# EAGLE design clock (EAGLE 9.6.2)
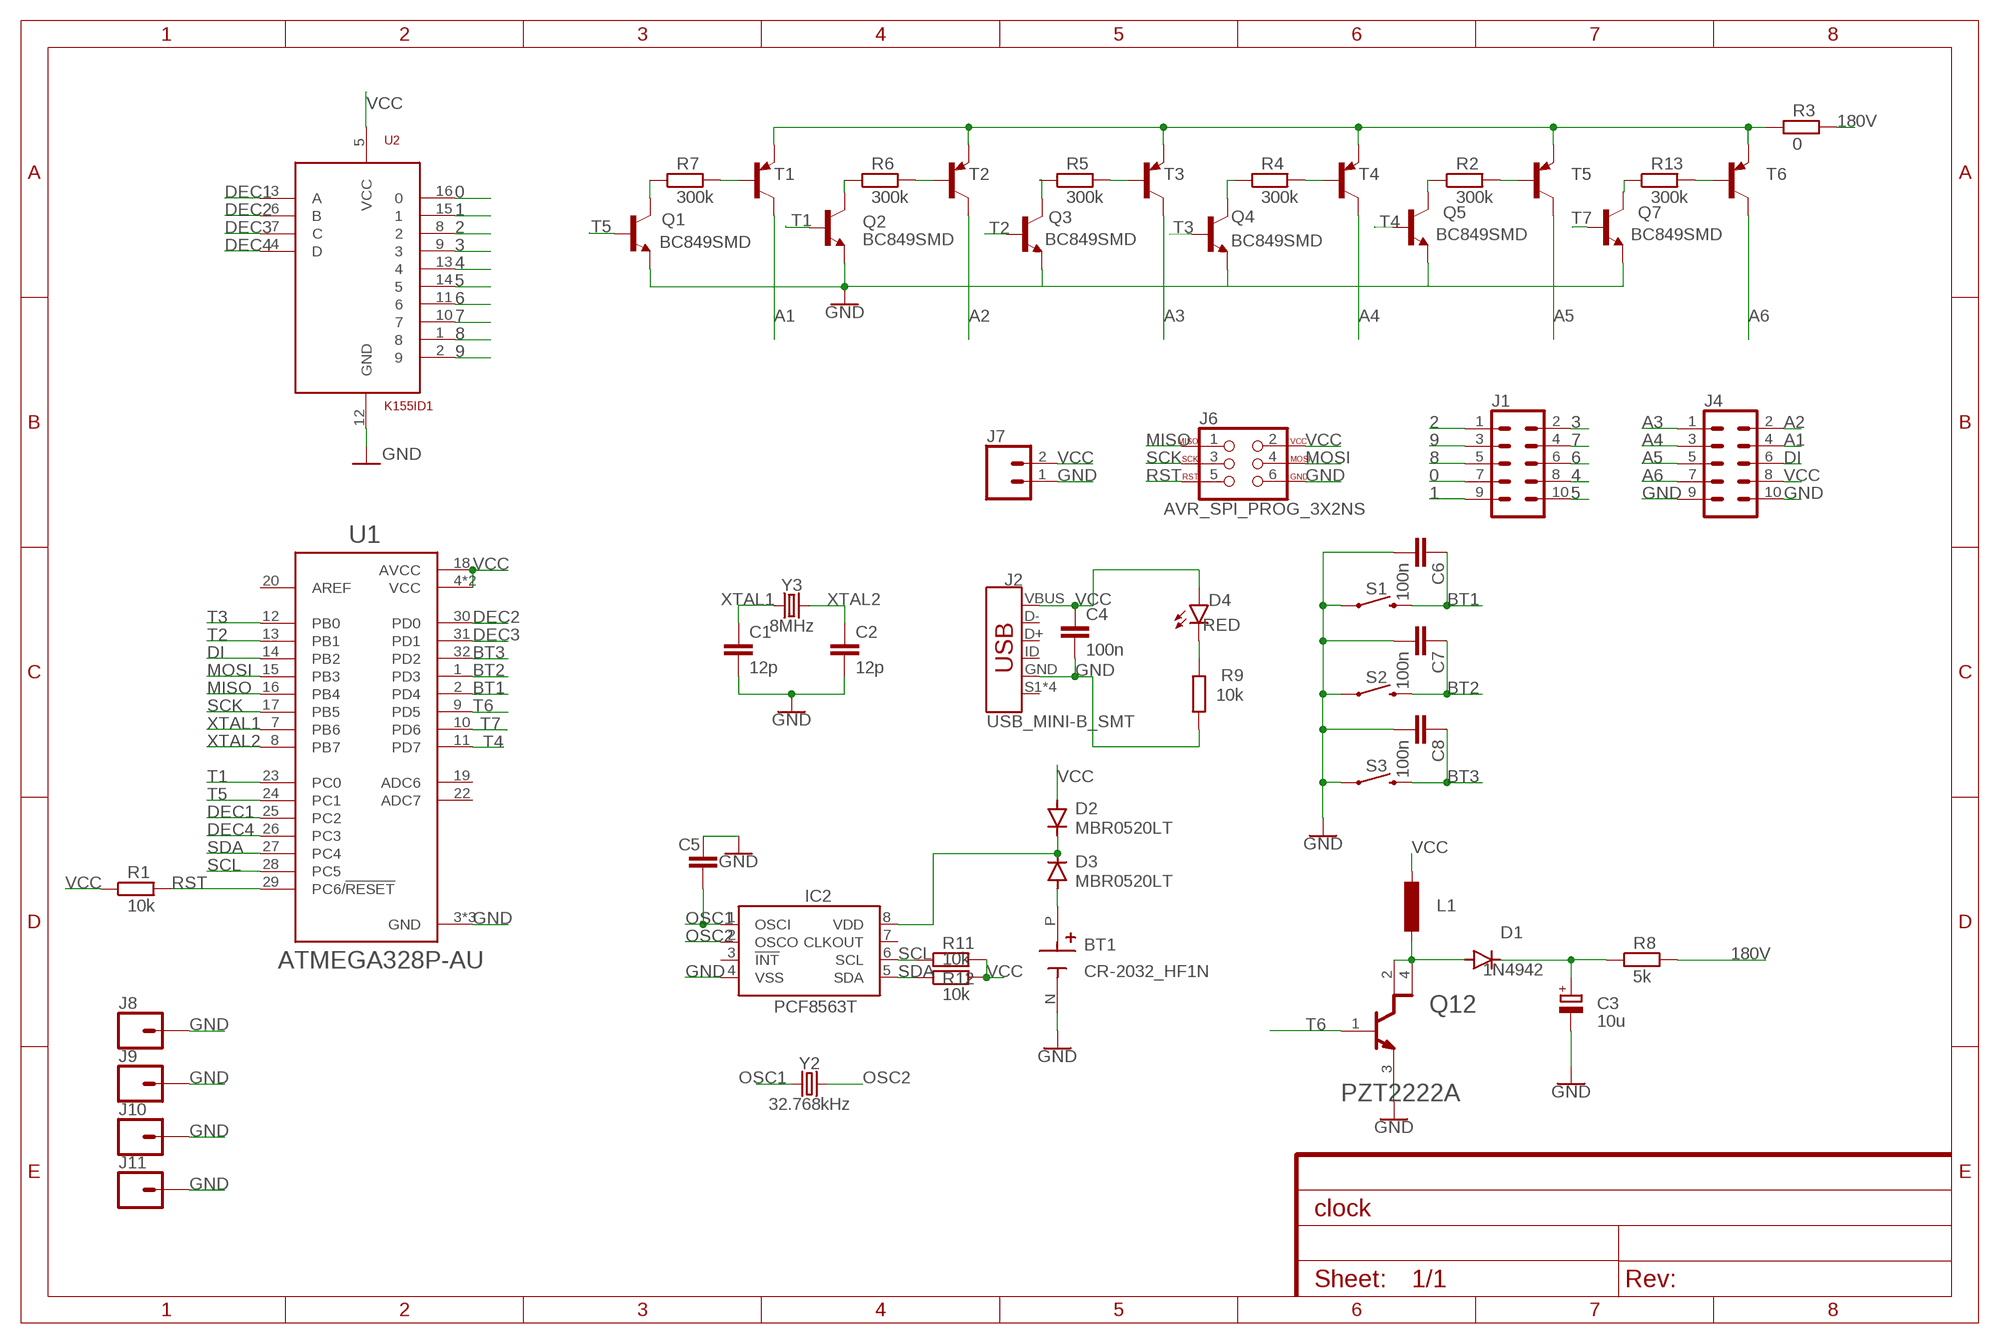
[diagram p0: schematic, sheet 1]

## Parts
BT1  CR-2032_HF1N  [BAT_CR-2032_HF1N]
C1  12p  C-EUC1206  [C1206]
C2  12p  C-EUC1206  [C1206]
C3  10u  CPOL-EUE3.5-10  [E3,5-10]
C4  100n  C-EUC1206  [C1206]
C5  C-EUC1206  [C1206]
C6  100n  C-EUC1206  [C1206]
C7  100n  C-EUC1206  [C1206]
C8  100n  C-EUC1206  [C1206]
D1  1N4942  [DO41-10]
D2  MBR0520LT  [SOD123]
D3  MBR0520LT  [SOD123]
D4  RED  LED-RED1206  [LED-1206]
IC2  PCF8563T  [SO8]
J1  CONN_05X2NO_SILK  [2X5_NOSILK]
J2  USB_MINI-B_SMT  [USB-MINIB]
J4  CONN_05X2NO_SILK  [2X5_NOSILK]
J6  AVR_SPI_PROG_3X2NS  [2X3-NS]
J7  CONN_021X02_NO_SILK  [1X02_NO_SILK]
J8  CONN_01PTH_2MM  [1X01_2MM]
J9  CONN_01PTH_2MM  [1X01_2MM]
J10  CONN_01PTH_2MM  [1X01_2MM]
J11  CONN_01PTH_2MM  [1X01_2MM]
L1  L-EU6000-XXX-RC  [6000-XXXX-RC]
Q1  BC849SMD  [SOT23-BEC]
Q2  BC849SMD  [SOT23-BEC]
Q3  BC849SMD  [SOT23-BEC]
Q4  BC849SMD  [SOT23-BEC]
Q5  BC849SMD  [SOT23-BEC]
Q7  BC849SMD  [SOT23-BEC]
Q12  ON_SEMI_PZT2222AON_SEMI_PZT2222A_0_0  [ON_SEMI_PZT2222A_0]
R1  10k  R-EU_R1206  [R1206]
R2  300k  R-EU_R1206  [R1206]
R3  0  R-EU_R1206  [R1206]
R4  300k  R-EU_R1206  [R1206]
R5  300k  R-EU_R1206  [R1206]
R6  300k  R-EU_R1206  [R1206]
R7  300k  R-EU_R1206  [R1206]
R8  5k  R-EU_R1206  [R1206]
R9  10k  R-EU_R1206  [R1206]
R11  10k  R-EU_R1206  [R1206]
R12  10k  R-EU_R1206  [R1206]
R13  300k  R-EU_R1206  [R1206]
S1  MOMENTARY-SWITCH-SPST-PTH-RIGHT-ANGLE-KIT  [TACTILE_SWITCH_PTH_RIGHT_ANGLE_KIT]
S2  MOMENTARY-SWITCH-SPST-PTH-RIGHT-ANGLE-KIT  [TACTILE_SWITCH_PTH_RIGHT_ANGLE_KIT]
S3  MOMENTARY-SWITCH-SPST-PTH-RIGHT-ANGLE-KIT  [TACTILE_SWITCH_PTH_RIGHT_ANGLE_KIT]
T1  BC807-16-PNP-SOT23-BEC  [SOT23-BEC]
T2  BC807-16-PNP-SOT23-BEC  [SOT23-BEC]
T3  BC807-16-PNP-SOT23-BEC  [SOT23-BEC]
T4  BC807-16-PNP-SOT23-BEC  [SOT23-BEC]
T5  BC807-16-PNP-SOT23-BEC  [SOT23-BEC]
T6  BC807-16-PNP-SOT23-BEC  [SOT23-BEC]
U1  ATMEGA328P-AU  [QFP80P900X900X120-32N]
U2  K155ID1  [DIP16-2.54-19.2X7.62MM]
Y2  32.768kHz  CRYSTAL-32.768KHZSMD-3.2X1.5  [CRYSTAL-SMD-3.2X1.5MM]
Y3  8MHz  CRYSTAL-8MHZSMD-HC49UP  [HC49UP]

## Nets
0: J1.7 U2.16
1: J1.9 U2.15
2: J1.1 U2.8
3: J1.2 U2.9
4: J1.8 U2.13
5: J1.10 U2.14
6: J1.6 U2.11
7: J1.4 U2.10
8: J1.5 U2.1
9: J1.3 U2.2
180V: R3.2 R8.2
A1: J4.4 T1.C
A2: J4.2 T2.C
A3: J4.1 T3.C
A4: J4.3 T4.C
A5: J4.5 T5.C
A6: J4.7 T6.C
BT1: C6.1 S1.2 U1.2(PD4)
BT2: C7.1 S2.2 U1.1(PD3)
BT3: C8.1 S3.2 U1.32(PD2)
DEC1: U1.25(PC2) U2.3(A)
DEC2: U1.30(PD0) U2.6(B)
DEC3: U1.31(PD1) U2.7(C)
DEC4: U1.26(PC3) U2.4(D)
DI: J4.6 U1.14(PB2)
GND: BT1.N(NEG) C1.2 C2.2 C3.- C4.2 C5.1 C6.2 C7.2 C8.2 IC2.4(VSS) J2.GND J4.9 J4.10 J6.6 J7.1 J8.1 J9.1 J10.1 J11.1 Q1.E Q2.E Q3.E Q4.E Q5.E Q7.E Q12.3(E) R9.1 S1.1 S2.1 S3.1 U1.3(GND) U1.5(GND) U1.21(GND) U2.12(GND)
MISO: J6.1 U1.16(PB4)
MOSI: J6.4 U1.15(PB3)
N$1: Q2.C R6.1
N$2: R7.2 T1.B
N$3: D1.A L1.2 Q12.2(1_C) Q12.4(2_C)
N$4: BT1.P(POS) D3.A
N$5: C3.+ D1.C R8.1
N$6: R6.2 T2.B
N$7: D4.C R9.2
N$8: Q3.C R5.1
N$9: R5.2 T3.B
N$10: Q1.C R7.1
N$11: Q4.C R4.1
N$13: Q5.C R2.1
N$14: R4.2 T4.B
N$15: R2.2 T5.B
N$16: R3.1 T1.E T2.E T3.E T4.E T5.E T6.E
N$17: D2.C D3.C IC2.8(VDD)
N$19: Q7.C R13.1
N$21: R13.2 T6.B
OSC1: C5.2 IC2.1(OSCI) Y2.P$1
OSC2: IC2.2(OSCO) Y2.P$2
RST: J6.5 R1.2 U1.29(PC6/!RESET)
SCK: J6.3 U1.17(PB5)
SCL: IC2.6(SCL) R11.1 U1.28(PC5)
SDA: IC2.5(SDA) R12.1 U1.27(PC4)
T1: Q2.B U1.23(PC0)
T2: Q3.B U1.13(PB1)
T3: Q4.B U1.12(PB0)
T4: Q5.B U1.11(PD7)
T5: Q1.B U1.24(PC1)
T6: Q12.1(B) U1.9(PD5)
T7: Q7.B U1.10(PD6)
VCC: C4.1 D2.A D4.A J2.VBUS J4.8 J6.2 J7.2 L1.1 R1.1 R11.2 R12.2 U1.4(VCC) U1.6(VCC) U1.18(AVCC) U2.5(VCC)
XTAL1: C1.1 U1.7(PB6) Y3.1
XTAL2: C2.1 U1.8(PB7) Y3.2
Unconnected: IC2.3(!INT!) IC2.7(CLKOUT) J2.D+ J2.D- J2.ID J2.S1(SHIELD) J2.S2(SHIELD) J2.S3(SHIELD) J2.S4(SHIELD) U1.19(ADC6) U1.20(AREF) U1.22(ADC7)

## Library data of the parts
BT1 = CR-2032_HF1N:CR-2032_HF1N: Check availability; AVAILABILITY: In Stock; CHECK_PRICES: https://www.snapeda.com/parts/CR-2032/HF1N/Panasonic/view-part/?ref=eda; DESCRIPTION: Coin, 20.0mm Lithium Manganese Dioxide 3 V Battery Non-Rechargeable (Primary); MF: Panasonic; MP: CR-2032/HF1N; PACKAGE: Package; PRICE: None; PURCHASE-URL: https://www.snapeda.com/api/url_track_click_mouser/?unipart_id=280179&manufacturer=Panasonic&part_name=CR-2032/HF1N&search_term=cr2032; SNAPEDA_LINK: https://www.snapeda.com/parts/CR-2032/HF1N/Panasonic/view-part/?ref=snap
C1 C2 C4-C8 = rcl:C-EU: CAPACITOR, European symbol; SPICEPREFIX: C
C3 = rcl:CPOL-EU: POLARIZED CAPACITOR, European symbol; SPICEPREFIX: C
D1 = diode:1N4942: DIODE
D2 D3 = diode:MBR0520LT: SCHOTTKY BARRIER RECTIFIER
D4 = SparkFun-LED:LED-RED: Red SMD LED; PROD_ID: DIO-09912
IC2 = PCF8563:PCF8563: Check availability; AVAILABILITY: Not in stock; DESCRIPTION: Real Time Clock (RTC) IC Clock/Calendar - I²C, 2-Wire Serial 8-TSSOP, 8-MSOP (0.118, 3.00mm Width); MF: NXP USA; MP: PCF8563; PACKAGE: Package; PRICE: None
J1 J4 = SparkFun-Connectors:CONN_05X2: Multi connection point. Often used as Generic Header-pin footprint for 0.1 inch spaced/style header connections For AVR SPI programming port, see special device with nice symbol: "AVR_SPI_PROG_5x2.dev" You can populate with any combo of single row headers, but if you'd like an exact match, check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
J2 = SparkFun-Connectors:USB_MINI-B: USB type Mini-B Connector Breaks out 5th pin, and includes shield pins if needed. SparkFun Products: SparkFun FTDI Basic Breakout SparkFun XBee Explorer USB SparkFun Redboard; PROD_ID: CONN-08193; SF_ID: PRT-00587
J6 = SparkFun-Connectors:AVR_SPI_PROG_3X2: AVR ISP 6 Pin This is the reduced ISP connector for AVR programming. Common on Arduino. This footprint will take up less PCB space and can be used with a 10-pin to 6-pin adapter such as SKU: BOB-08508 **Special note about "TEST_POINT" package. The stop mask is on the top side, so if you want your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
J7 = SparkFun-Connectors:CONN_02: Multi connection point. Often used as Generic Header-pin footprint for 0.1 inch spaced/style header connections
J8-J11 = SparkFun-Connectors:CONN_01: Single connection point. Often used as Generic Header-pin footprint for 0.1 inch spaced/style header connections
L1 = rcl:L-EU: INDUCTOR, European symbol; SPICEPREFIX: L
Q1-Q5 Q7 = transistor-npn:BC849*: NPN Transistor
Q12 = ON Semi - PZT2222A:ON_SEMI_PZT2222A: TRANS NPN 40V 1A SOT-223; CENTROID_NOT_SPECIFIED: No; DATASHEET: https://www.fairchildsemi.com/datasheets/PZ/PZT2222A.pdf; DIGIKEY_DESCRIPTION: TRANS NPN 40V 1A SOT-223; DIGIKEY_PART_NUMBER: PZT2222ACT-ND; LEAD_FREE: yes; MF: ON Semi; MFG_PACKAGE_IDENT: CASE 318E−04; MOUSER_PART_NUMBER: 512-PZT2222A; MPN: PZT2222A; PACKAGE: SOT223; PREFIX: Q; ROHS: yes; TEMPERATURE_RANGE_HIGH: +150°C; TEMPERATURE_RANGE_LOW: -55°C
R1-R9 R11-R13 = rcl:R-EU_: RESISTOR, European symbol; SPICEPREFIX: R
S1-S3 = SparkFun-Switches:MOMENTARY-SWITCH-SPST: Momentary Switch (Pushbutton) - SPST; PROD_ID: CONN-10672; SF_SKU: COM-10791
T1-T6 = transistor:*-PNP-: PNP Transistror
U1 = ATMEGA328P-AU:ATMEGA328P-AU: ATmega Series 20 MHz 32 KB Flash 2 KB SRAM 8-Bit Microcontroller - TQFP-32 Check availability; AVAILABILITY: In Stock; DESCRIPTION: AVR AVR® ATmega Microcontroller IC 8-Bit 20MHz 32KB (16K x 16) FLASH 32-TQFP (7x7); MF: Microchip Technology; MP: ATMEGA328P-AU; PACKAGE: TQFP-32 Microchip; PRICE: None; PURCHASE-URL: https://pricing.snapeda.com/search/part/ATMEGA328P-AU/?ref=eda
U2 = TimeExpander:K155ID1: Soviet version of SN74141 BCD to Decimal Decoder / Nixie Driver
Y2 = SparkFun-Clocks:CRYSTAL-32.768KHZ: 32.768kHz Crystal; PROD_ID: XTAL-13062
Y3 = SparkFun-Clocks:CRYSTAL-8MHZ: 8MHz Crystal; PROD_ID: XTAL-11706

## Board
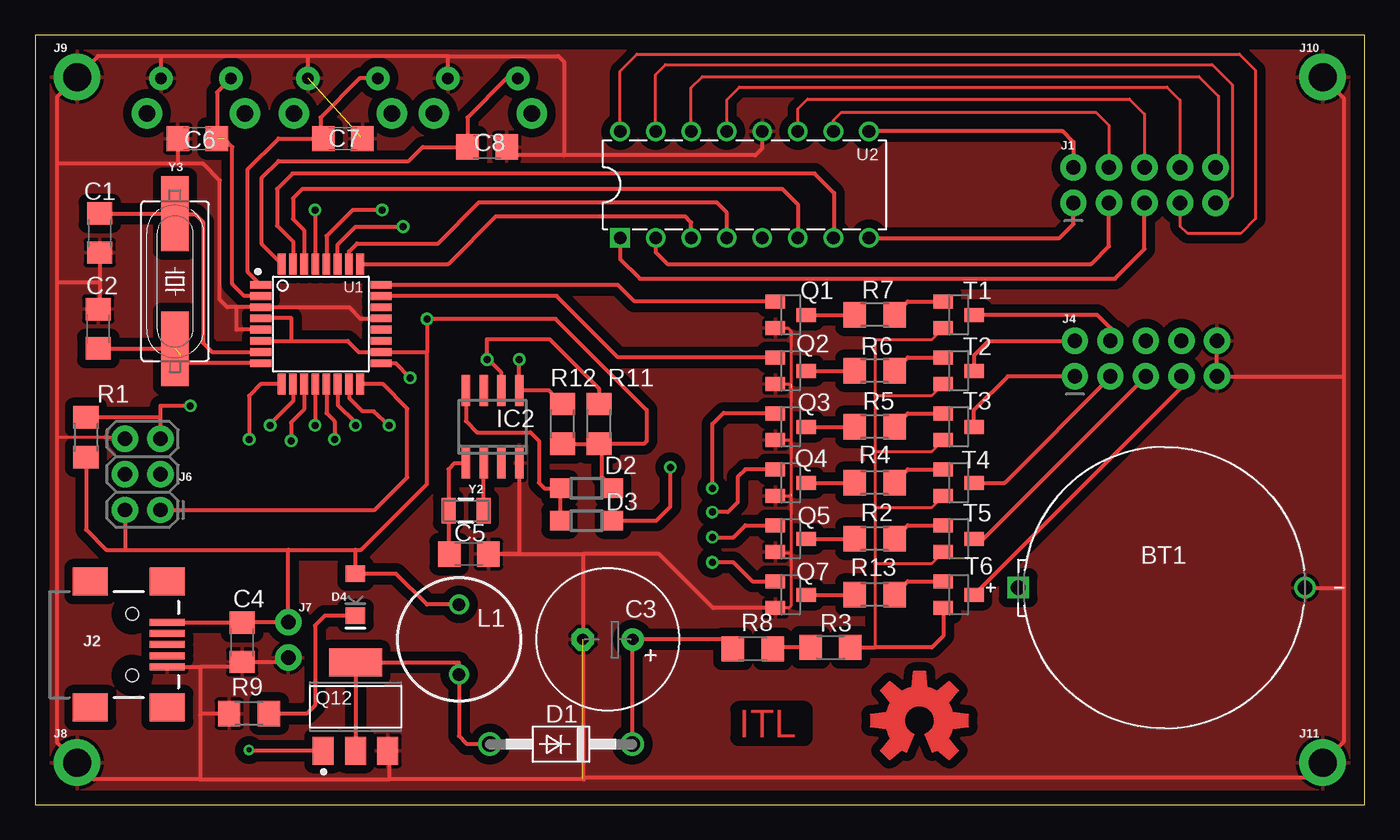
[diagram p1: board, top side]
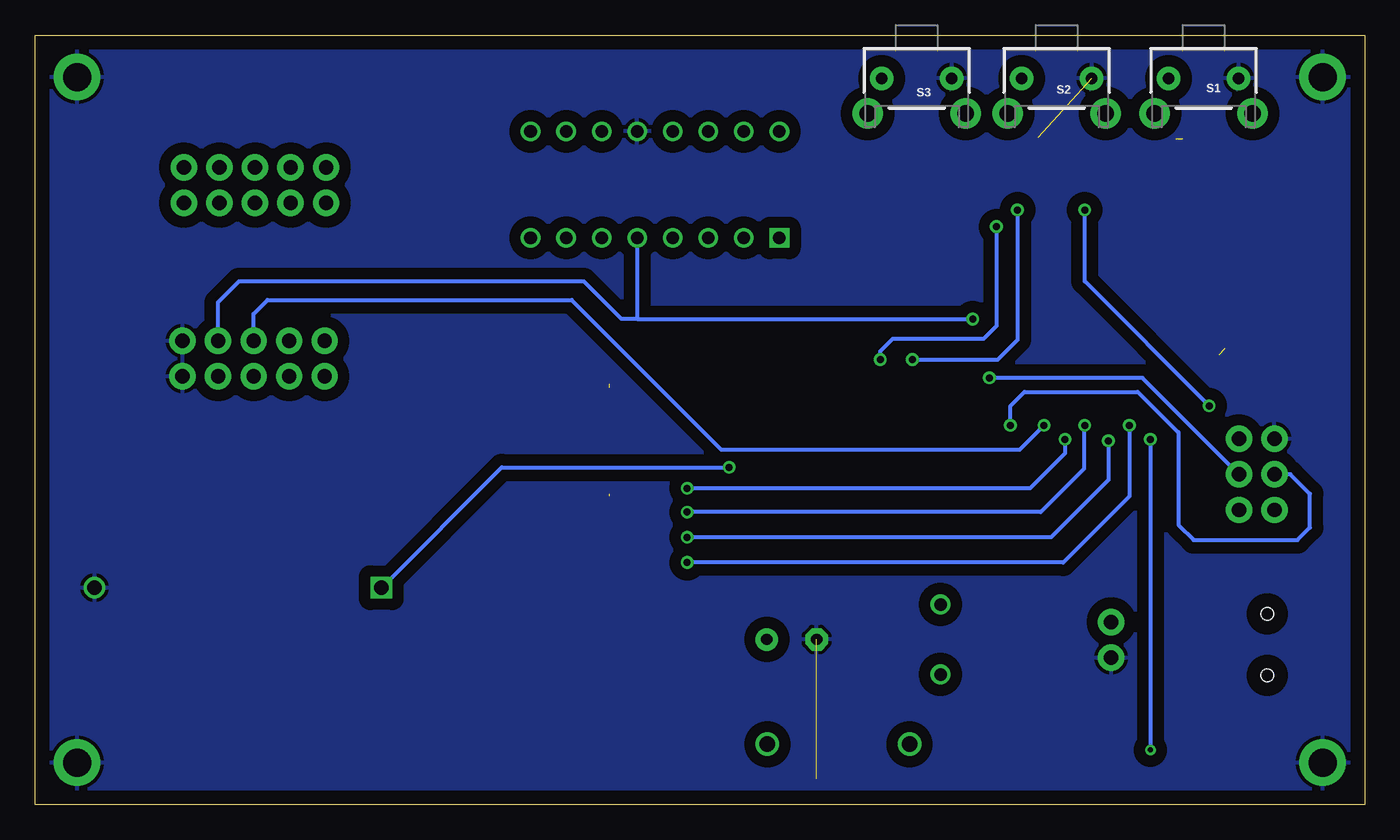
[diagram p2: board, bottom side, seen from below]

Size 95 x 55 mm. Coordinates in mm from the lower left corner, seen from the top.
Outline: 0,0 95,0 95,55 0,55 0,0
Copper layers (1*16): Top 0.035mm / dielectric 1.5mm / Bottom 0.035mm
Design rules "default": minimum track width 6mil, minimum drill 0.35mm, track to track 6mil, track to pad 6mil, pad to pad 6mil, via to via 6mil, smd to smd 6mil, copper to edge 40mil, drill to drill 6mil, minimum pad ring 10mil, minimum via ring 8mil, stop-mask expansion 4mil, vias tented up to drill 0mil, thermal gap 10mil

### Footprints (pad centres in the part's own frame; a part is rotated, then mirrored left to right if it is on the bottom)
BAT_CR-2032_HF1N = drill 1.04: N -10.05,0 | drill 1.04 square: P 10.45,0
C1206 = smd 1.6 x 1.8: 1 -1.4,0; 2 1.4,0
E3,5-10 = drill 0.813 pad 1.6: + -1.778,0 | drill 0.813 pad 1.6 octagon: - 1.778,0
DO41-10 = drill 1.118: A 5.08,0; C -5.08,0
SOD123 = smd 1.4 x 1.4: A 1.9,0; C -1.9,0
LED-1206 = smd 1.2 x 1.4: A -1.5,0; C 1.5,0
SO8 = smd 0.6 x 2.2: 1 -1.905,-2.6; 2 -0.635,-2.6; 3 0.635,-2.6; 4 1.905,-2.6; 5 1.905,2.6; 6 0.635,2.6; 7 -0.635,2.6; 8 -1.905,2.6
2X5_NOSILK = drill 1.016 pad 1.88: 1 0,0; 2 0,2.54; 3 2.54,0; 4 2.54,2.54; 5 5.08,0; 6 5.08,2.54; 7 7.62,0; 8 7.62,2.54; 9 10.16,0; 10 10.16,2.54
USB-MINIB = smd 2.5 x 0.5: D+ 2.5,0; D- 2.5,0.8; GND 2.5,-1.6; ID 2.5,-0.8; VBUS 2.5,1.6 | smd 2.5 x 2: S1 -3,4.5; S2 2.5,4.5; S3 -3,-4.5; S4 2.5,-4.5 | hole 0.9: 0,2.2; 0,-2.2
2X3-NS = drill 1.016 pad 1.88: 1 -2.54,-1.27; 2 -2.54,1.27; 3 0,-1.27; 4 0,1.27; 5 2.54,-1.27; 6 2.54,1.27
1X02_NO_SILK = drill 1.016 pad 1.88: 1 0,0; 2 2.54,0
1X01_2MM = drill 2 pad 3.302: 1 0,0
6000-XXXX-RC = drill 0.9 pad 1.422: 1 -2.5,0; 2 2.5,0
SOT23-BEC = smd 1 x 1.4: B -0.95,-1.1; C 0,1.1; E 0.95,-1.1
ON_SEMI_PZT2222A_0 = smd 1.5 x 2: 1 -2.3,-3.15; 2 0,-3.15; 3 2.3,-3.15 | smd 3.8 x 2: 4 0,3.15
R1206 = smd 1.6 x 1.803: 1 -1.422,0; 2 1.422,0
TACTILE_SWITCH_PTH_RIGHT_ANGLE_KIT = drill 0.8 pad 1.7: 1 -2.5,0; 2 2.5,0 | drill 1.2 pad 2.2: ANCHOR1 -3.5,2.5; ANCHOR2 3.5,2.5
QFP80P900X900X120-32N = smd 1.5 x 0.55: 1 -4.3,2.8; 2 -4.3,2; 3 -4.3,1.2; 4 -4.3,0.4; 5 -4.3,-0.4; 6 -4.3,-1.2; 7 -4.3,-2; 8 -4.3,-2.8; 17 4.3,-2.8; 18 4.3,-2; 19 4.3,-1.2; 20 4.3,-0.4; 21 4.3,0.4; 22 4.3,1.2; 23 4.3,2; 24 4.3,2.8 | smd 0.55 x 1.5: 9 -2.8,-4.3; 10 -2,-4.3; 11 -1.2,-4.3; 12 -0.4,-4.3; 13 0.4,-4.3; 14 1.2,-4.3; 15 2,-4.3; 16 2.8,-4.3; 25 2.8,4.3; 26 2,4.3; 27 1.2,4.3; 28 0.4,4.3; 29 -0.4,4.3; 30 -1.2,4.3; 31 -2,4.3; 32 -2.8,4.3
DIP16-2.54-19.2X7.62MM = drill 0.9 pad 1.4 square: 1 -8.89,-3.81 | drill 0.9 pad 1.4: 2 -6.35,-3.81; 3 -3.81,-3.81; 4 -1.27,-3.81; 5 1.27,-3.81; 6 3.81,-3.81; 7 6.35,-3.81; 8 8.89,-3.81; 9 8.89,3.81; 10 6.35,3.81; 11 3.81,3.81; 12 1.27,3.81; 13 -1.27,3.81; 14 -3.81,3.81; 15 -6.35,3.81; 16 -8.89,3.81
CRYSTAL-SMD-3.2X1.5MM = smd 1 x 1.8: P$1 -1.25,0; P$2 1.25,0
HC49UP = smd 5.334 x 1.93: 1 -4.826,0; 2 4.826,0

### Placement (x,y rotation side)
BT1  80.7,15.5 180 top
C1  4.62,40.85 270 top
C2  4.52,34 90 top
C3  40.93,11.8 180 top
C4  14.8,11.6 270 top
C5  31,17.9 180 top
C6  11.6,47.6 180 top
C7  22,47.6 0 top
C8  32.3,47 0 top
D1  37.59,4.31 180 top
D2  39.4,22.6 0 top
D3  39.4,20.3 0 top
D4  22.9,15 270 top
IC2  32.7,27 0 top
J1  74.2,43 0 top
J2  6.95,11.43 0 top
J4  74.3,30.6 0 top
J6  7.7,23.6 90 top
J7  18.1,10.5 90 top
J8  3,3 0 top
J9  3,52 0 top
J10  92,52 0 top
J11  92,3 0 top
L1  30.3,11.8 270 top
Q1  54,35 270 top
Q2  54,31 270 top
Q3  54,27 270 top
Q4  54,23 270 top
Q5  54,19 270 top
Q7  54,15 270 top
Q12  22.9,7 0 top
R1  3.65,26.25 90 top
R2  60,19 0 top
R3  56.84,11.23 180 top
R4  60,23 0 top
R5  60,27 0 top
R6  60,31 0 top
R7  60,35 0 top
R8  51.29,11.13 0 top
R9  15.3,6.5 0 top
R11  40.3,27.2 270 top
R12  37.7,27.2 270 top
R13  60,15 0 top
S1  11.5,51.9 180 bottom
S2  22,51.9 180 bottom
S3  32,51.9 180 bottom
T1  66,35 270 top
T2  66,31 270 top
T3  66,27 270 top
T4  66,23 270 top
T5  66,19 270 top
T6  66,15 270 top
U1  20.43,34.34 0 top
U2  50.7,44.3 0 top
U$1  [OSHW-LOGO-L_COPPER]  63.2,6 0 top
Y2  30.8,21 0 top
Y3  10,37.4 270 top

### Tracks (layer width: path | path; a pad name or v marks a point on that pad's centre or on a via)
0
  Top 0.2: J1.7 81.82,41.35 82.37,40.81 86.15,40.81 87.2,41.86 87.2,52.48 86.06,53.63 43.01,53.63 41.81,52.43 U2.16
1
  Top 0.2: J1.9 85.11,43 85.55,43.45 85.55,51.43 84.11,52.88 45.05,52.88 44.35,52.18 U2.15
2
  Top 0.3: U2.8 73.2,40.49 74.2,41.49 J1.1
3
  Top 0.3: U2.9 73.43,48.11 74.2,47.34 J1.2
4
  Top 0.2: J1.8 81.82,50.34 80.89,51.27 50.33,51.27 49.43,50.37 U2.13
5
  Top 0.2: J1.10 84.56,45.74 84.56,50.64 83.18,52.02 47.69,52.02 46.89,51.22 U2.14
6
  Top 0.2: J1.6 79.28,49.34 78.2,50.42 55.21,50.42 54.51,49.72 U2.11
7
  Top 0.2: J1.4 76.74,48.54 75.81,49.47 57.61,49.47 57.05,48.91 U2.10
8
  Top 0.3: U2.1 41.81,38.99 43.22,37.58 77.16,37.58 79.28,39.7 J1.5
9
  Top 0.3: U2.2 44.35,39.48 45.19,38.63 75.47,38.63 76.74,39.9 J1.3
180V
  Top 0.3: R8.2 52.81,11.23 R3.2
A1
  Top 0.3: J4.4 76.84,34.06 75.9,35 T1.C
A2
  Top 0.3: J4.2 68.14,33.14 67.1,32.1 T2.C
A3
  Top 0.3: J4.1 69.5,30.6 67.1,28.2 T3.C
A4
  Top 0.3: J4.3 76.84,30.54 69.3,23 T4.C
A5
  Top 0.3: J4.5 67.78,19 T5.C
A6
  Top 0.3: J4.7 81.92,29.82 T6.C
BT1  (1 unrouted)
  Top 0.3: 16.11,36.36 U1.2 14.96,36.34 14.1,37.2 14.1,47 13.5,47.6 | S1.2 13,50.9 C6.1
BT2
  Top 0.3: U1.1 15.2,38.07 15.2,45.4 17.4,47.6 20.4,47.6 | 20.4,47.6 C7.1 | S2.2 23.2,51.9 20.4,49.1 20.4,47.6
BT3
  Top 0.3: C8.1 31,47.1 | U1.32 16.2,40.07 16.2,44.8 17.4,46 26.7,46 27.7,47 C8.1 | S3.2 33.7,51.9 30.9,49.1 C8.1
DEC1
  Top 0.3: U2.3 46.89,41.59 46.44,42.04 32.94,42.04 29.54,38.64 U1.25 23.13,38.74
DEC2
  Top 0.3: U2.6 54.51,42.89 53.4,44 19.1,44 18.43,43.33 18.43,41.84 19.23,41.04 U1.30
DEC3
  Top 0.3: U2.7 57.1,40.54 57.1,43.7 55.7,45.1 18.4,45.1 17.3,44 17.3,41.37 18.43,40.24 U1.31
DEC4
  Top 0.3: U2.4 49.43,42.29 48.68,43.04 31.73,43.04 28.79,40.1 23,40.1 22.43,39.53 U1.26 22.45,38.66
DI  (via drill 0.5)
  Top 0.3: U1.14 21.63,28.57 22.9,27.3 v22.9,27.1
  Bottom 0.3: J4.6 79.38,35.06 78.38,36.06 56.65,36.06 45.93,25.34 24.66,25.34 v22.9,27.1
GND  (4 unrouted)
  Top 0.2: J6.6 6.33,26.24 1.6,26.24 | Q1.E 53.8,34.05 54,33.85 54,30.1 | 54,30.1 54,29.8 | 54,30.05 54,26 | 54,26 54,22.05 | 54,22.2 54,22 | 54,22 54,18 | 54,18 54,14.2 53.85,14.05 Q7.E | Q5.E 52.95,18 54,18 | Q3.E 53.95,26.05 54,26 | Q2.E 53.95,30.05 54,30.1 | Q4.E 53.95,22.05 54,22
  Top 0.3: J2.GND 11.8,9.83 | 25.17,34.8 25.11,34.74 U1.21 24.7,34.71 23.27,34.71 22.45,35.54 U1.3 14.44,35.54 | U1.5 14.4,33.94 14.4,35.5 14.44,35.54 | 14.44,35.54 13.74,35.54 13.2,36.08 13.2,44.6 12,45.8 10.2,45.8 | 11.8,9.83 11.8,6.4 | 11.8,6.4 11.8,1.8 | 1.6,37.3 1.6,26.24 1.6,4.4 J8.1 4.2,1.8 11.8,1.8 | 1.6,37.3 1.6,45.8 | 1.6,45.8 1.6,50.6 J9.1 4.5,53.5 9,53.5 | 11.8,1.8 25.3,1.8 | J10.1 93.5,50.5 93.5,30.6 | 93.5,30.6 93.5,15.5 | 93.5,15.5 93.5,4.5 J11.1 90.9,1.9 39.15,1.9 C3.- 39.15,17.9 | IC2.4 34.6,17.9 C5.1 39.15,17.9 | Q12.3 25.3,3.75 25.3,1.8 | 29.5,53.5 19.5,53.5 | 19.5,53.5 9,53.5 | J4.10 J4.9 93.5,30.6 | J7.1 17.8,10.2 C4.2 14.43,9.83 11.8,9.83 | 10.2,45.8 1.6,45.8 | C1.2 4.62,37.3 | 4.62,37.3 4.62,35.5 C2.2 | 4.62,37.3 1.6,37.3 | 33.3,47 C8.2 34.29,46.41 37.8,46.41 | 37.8,46.41 51.47,46.41 51.97,46.91 U2.12 | C6.2 10.2,45.8 | R9.1 11.9,6.5 11.8,6.4 | Q7.E 48.45,14.05 44.6,17.9 39.15,17.9 | 25.3,1.8 39.2,1.8 39.15,1.85 | C7.2 23.3,47.7 | S1.1 9,53.5 | S2.1 19.5,53.5 | S3.1 29.5,53.5 | 37.8,46.41 37.8,53.1 37.4,53.5 29.5,53.5 | BT1.N 93.5,15.5
  pour Bottom (isolate 0.813): 0,0.3 0,54.7 0.2,54.9 95.1,54.9 95.1,0.4 94.7,0 0.3,0
  pour Top (isolate 0.61): 0,0 0,55 95,55 95,0.1 94.9,0
MISO
  Top 0.3: J6.1 24.27,21.06 26.6,23.39 26.6,28.3 24.86,30.04 U1.16
MOSI  (via drill 0.5)
  Top 0.3: v25.3,27.1 24.2,28.1 23.4,28.1 22.46,29.04 22.46,30.01 U1.15
  Bottom 0.3: v25.3,27.1 25.3,28.5 24.3,29.5 16.2,29.5 13.3,26.6 13.3,20 12.2,18.9 4.8,18.9 3.9,19.8 3.9,22.2 5.3,23.6 J6.4
N$1
  Top 0.3: Q2.C R6.1
N$2
  Top 0.3: R7.2 62.37,35.95 T1.B
N$3
  Top 0.3: D1.A 30.89,4.31 30.3,4.9 L1.2 30.3,10.15 Q12.4 Q12.2
N$4  (via drill 0.5)
  Top 0.3: D3.A 44.4,20.3 45.4,21.3 v45.4,24.1
  Bottom 0.3: BT1.P 61.65,24.1 v45.4,24.1
N$5
  Top 0.3: D1.C 42.67,11.76 C3.+ 49.5,11.8 49.87,11.43 R8.1
N$6
  Top 0.3: R6.2 62.37,31.95 T2.B
N$7
  Top 0.3: D4.C 20.7,13.5 20,12.8 20,7.1 19.4,6.5 R9.2
N$8
  Top 0.3: Q3.C R5.1
N$9
  Top 0.3: R5.2 62.37,27.95 T3.B
N$10
  Top 0.3: Q1.C R7.1
N$11
  Top 0.3: Q4.C R4.1
N$13
  Top 0.3: Q5.C R2.1
N$14
  Top 0.3: R4.2 62.37,23.95 T4.B
N$15
  Top 0.3: R2.2 62.37,19.95 T5.B
N$16
  Top 0.2: T1.E 64.05,33.2 60,33.2 60,29.2 | 60,29.2 60,25.2 | 60,25.2 60,21.2 | 60,21.2 60,17.2 | 60,17.2 60,11.23 | T2.E 64.05,29.2 60,29.2 | T3.E 64.05,25.2 60,25.2 | T4.E 64.05,21.2 60,21.2 | T5.E 64.05,17.2 60,17.2
  Top 0.3: R3.1 60,11.23 64.08,11.23 64.9,12.05 T6.E
N$17
  Top 0.3: D3.C D2.C 36.4,22.6 36,23 36,26 35.4,26.6 31.6,26.6 30.8,27.41 IC2.8
N$19
  Top 0.3: Q7.C R13.1
N$21
  Top 0.3: R13.2 62.37,15.95 T6.B
OSC1
  Top 0.3: Y2.P$1 29.59,21.05 | Y2.P$1 29.55,23.95 30,24.4 IC2.1 | C5.2 29.6,20.95 Y2.P$1
OSC2
  Top 0.3: Y2.P$2 32.06,21.02 IC2.2
RST  (via drill 0.5)
  Top 0.3: R1.2 8.97,27.67 J6.5 8.97,28.5 v11.1,28.5 | U1.29 20,38.67 v20,42.5
  Bottom 0.3: v11.1,28.5 20,37.4 v20,42.5
SCK  (via drill 0.5)
  Top 0.3: U1.17 25.76,31.54 v26.8,30.5
  Bottom 0.3: J6.3 15.87,30.5 v26.8,30.5
SCL  (via drill 0.5)
  Top 0.3: U1.28 20.83,40.63 22.7,42.5 v24.8,42.5 | v32.3,31.8 32.3,31.9 | 32.3,31.9 32.3,33.26 36.77,33.26 40.3,29.72 R11.1 | IC2.6 33.34,30.86 32.3,31.9
  Bottom 0.3: v24.8,42.5 24.8,33.2 26.2,31.8 v32.3,31.8
SDA  (via drill 0.5)
  Top 0.3: U1.27 21.63,40.03 22.9,41.3 v26.3,41.3 | v34.6,31.8 IC2.5 36.72,29.6 R12.1
  Bottom 0.3: v34.6,31.8 34.6,32.4 33.7,33.3 27.2,33.3 26.3,34.2 v26.3,41.3
T1
  Top 0.3: U1.23 37.28,36.34 41.67,31.95 Q2.B
T2  (via drill 0.5)
  Top 0.3: U1.13 20.83,27.97 21.4,27.4 v21.4,26.1 | v48.4,22.6 48.4,27.2 49.2,28 52.85,28 Q3.B
  Bottom 0.3: v21.4,26.1 21.4,25.1 23.9,22.6 v48.4,22.6
T3  (via drill 0.5)
  Top 0.2: 20.03,27.23 v20,27.1
  Top 0.3: U1.12 20.03,27.23 | Q4.B 50.75,23.95 50.2,23.4 50.2,21.6 49.5,20.9 v48.4,20.9
  Bottom 0.3: v20,27.1 20.04,27.16 20.04,23.99 23.13,20.9 v48.4,20.9
T4  (via drill 0.5)
  Top 0.3: U1.11 19.23,28.23 18.3,27.3 v18.3,26 | v48.4,19.1 49.9,19.1 50.75,19.95 Q5.B
  Bottom 0.3: v18.3,26 18.3,23.2 22.4,19.1 v48.4,19.1
T5
  Top 0.3: U1.24 41.66,37.14 42.85,35.95 Q1.B
T6  (via drill 0.35, 0.5)
  Top 0.3: v15.3,26.1 15.3,29.2 16.14,30.04 U1.9 | Q12.1 15.3,3.85 v15.3,3.9
  Bottom 0.3: v15.3,26.1 v15.3,3.9
T7  (via drill 0.5)
  Top 0.3: U1.10 18.43,28.83 16.8,27.2 v16.8,27.1 | v48.4,17.3 49.9,17.3 51.25,15.95 Q7.B
  Bottom 0.3: v16.8,27.1 16.8,22.03 21.53,17.3 v48.4,17.3
VCC  (via drill 0.5)
  Top 0.3: U1.6 18.3,33.14 | 18.3,33.14 22.35,33.14 23.18,32.31 24.7,32.31 U1.18 24.77,32.3 28,32.3 | U1.4 16.19,34.8 18.3,34.8 18.3,33.14 | 3.68,24.86 R1.1 3.65,19.65 5.1,18.2 6.43,18.2 | 28,32.3 28,22.9 23.3,18.2 22.9,18.2 | 6.43,18.2 18.1,18.2 | 18.1,18.2 22.9,18.2 | J6.2 6.43,18.2 | 28,32.3 v28,34.7 37.2,34.7 43.7,28.2 43.7,25.98 43.5,25.78 40.5,25.78 | R12.2 R11.2 40.5,25.78 | D2.A 40.5,23.4 40.5,25.78 | J2.VBUS 14.77,13.03 C4.1 14.84,13.04 J7.2 18.1,18.2 | 22.9,18.2 D4.A 25.8,16.5 28,14.3 L1.1
  Bottom 0.3: 51.97,34.7 v28,34.7 | U2.5 51.97,34.7 | 51.97,34.7 53.1,34.7 55.8,37.4 80.42,37.4 81.92,35.9 J4.8
XTAL1
  Top 0.3: Y3.1 10.05,42.18 10.1,42.18 | 10.1,42.18 11.45,42.18 12,41.63 12,33 12.66,32.34 U1.7 | C1.1 10.03,42.25 10.1,42.18
XTAL2  (2 unrouted)
  Top 0.3: 16.11,31.52 U1.8 10.86,31.54 9.8,32.6 | 10.42,32.12 10.44,32.14 | C2.1 9.8,32.6 | 9.8,32.6 9.97,32.6

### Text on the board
Top: ITL

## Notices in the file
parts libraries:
SparkFun-Aesthetics: Licensing: Creative Commons ShareAlike 4.0 International - https://creativecommons.org/licenses/by-sa/4.0
